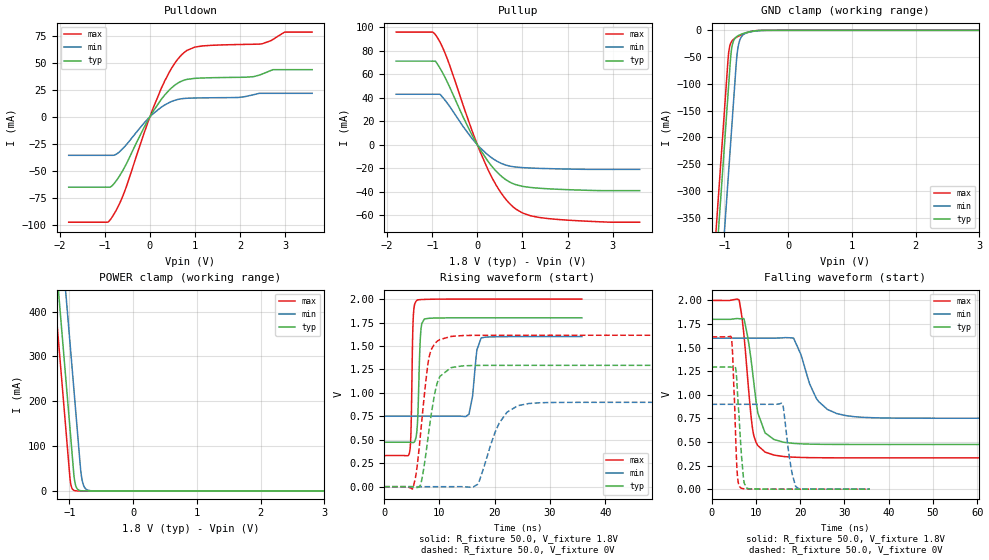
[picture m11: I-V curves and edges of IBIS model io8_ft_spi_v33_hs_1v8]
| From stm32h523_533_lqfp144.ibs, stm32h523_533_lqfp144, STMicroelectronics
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[Model]   io8_ft_spi_v33_hs_1v8
Model_type I/O
Polarity   Non-Inverting
Enable   Active-Low
| CAP_THRESHOLD on pad IOFT is "UDTCAPC" :
| Rising=20.0% of vddiom   Falling=80.0% of vddiom
| C_comp min and max val. don't necessarily correlate with the min and max pvt
| but are the smallest and greatest pad capacitance found.
| var   typ   min   max
C_comp   3.69208pF  3.66960pF  3.86716pF
|C_comp_pullup   2.28930pF  2.21680pF  2.21510pF
|C_comp_pulldown   1.40278pF  1.45280pF  1.65206pF
Vinl = 480.0mV
Vinh = 1.4V
Vmeas = 900.0mV   | Reference voltage for timing measurements
Cref  = 50.0pF   | Timing specification test load capacitance value
Rref  = 100.0MOhm   | Timing specification test load resistance value
Vref  = 900.0mV   | Timing specification test load voltage
[Model Spec]
| TIME_THRESHOLD on pin ZIV33M is "CMOS" :
| Rising=40.0% of vddiom   Falling=60.0% of vddiom
Vinl 693.80000mV 621.80000mV 774.80000mV
Vinh 1.05820V 933.20000mV 1.16320V
| variable   typ   min   max
[Temperature Range] 25.0 125.0 -40.0
| variable   typ   min   max
[Voltage Range] 1.8V 1.6V 2.0V
| variable   typ   min   max
[POWER Clamp Reference] 1.8V 1.6V 2.0V
| variable   typ   min   max
[GND Clamp Reference] 0V 0V 0V
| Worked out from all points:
|   slope of the pulldown table from 0 to 0.27 V, typ, clamps not added: 15.8 ohm
|   slope of the pullup table from 0 to 0.27 V, typ, clamps not added: 17.1 ohm
|   GND clamp passes 1 mA (typ) near -0.52 V on its own axis
|   POWER clamp passes 1 mA (typ) near -0.84 V on its own axis
|   rising waveform, R_fixture 50.0, V_fixture 1.8V: 20-80 % time 426ps typ, 879ps min, 294ps max; typ from 0.474 V to 1.8 V
|   falling waveform, R_fixture 50.0, V_fixture 1.8V: 20-80 % time 2.56ns typ, 4.2ns min, 1.95ns max; typ from 1.8 V to 0.474 V
|   rising waveform, R_fixture 50.0, V_fixture 0V: 20-80 % time 1.97ns typ, 3.43ns min, 1.71ns max; typ from 0 V to 1.29 V
|   falling waveform, R_fixture 50.0, V_fixture 0V: 20-80 % time 1.1ns typ, 1.55ns min, 755ps max; typ from 1.29 V to 0 V
[POWER Clamp]
-1.8V     1.518A     1.709A     1.407A
-1.23V    548.8mA    740.2mA    437.5mA
-1.16V    429.8mA    621.2mA    318.5mA
-1.05V    242.8mA    434.2mA    131.5mA
-980mV    123.8mA    315.2mA    17.95mA
-930mV    38.81mA    230.2mA    1.49mA
-910mV    17.82mA    196.2mA    550.8uA
-890mV    8.18mA     162.2mA    203.5uA
-810mV    363.5uA    33.6mA     3.797uA
-770mV    76.62uA    10.47mA    518.8nA
-710mV    7.416uA    1.822mA    26.34nA
3.6V      0A         0A         0A
[GND Clamp]
-1.8V     -1.579A    -1.74A     -1.515A
-1.24V    -627.3mA   -788.3mA   -562.7mA
-1.05V    -304.3mA   -465.3mA   -239.7mA
-940mV    -117.3mA   -278.3mA   -52.69mA
-930mV    -100.3mA   -261.3mA   -40.52mA
-900mV    -50.11mA   -210.3mA   -24.23mA
-880mV    -30.95mA   -176.3mA   -20.02mA
-810mV    -12.18mA   -57.97mA   -13.23mA
-780mV    -9.807mA   -29.1mA    -11.19mA
-690mV    -5.41mA    -7.142mA   -6.184mA
-420mV    -170.4uA   -446.1uA   -81.94uA
3.6V      5.755nA    953.4nA    228.2pA
| variable   typ   min   max
[Pullup Reference] 1.8V 1.6V 2.0V
| variable   typ   min   max
[Pulldown Reference] 0V 0V 0V
[Pullup]
-1.8V     71.25mA    43.04mA    95.97mA
-990mV    71.25mA    43.04mA    95.97mA
-900mV    69.58mA    43.04mA    92.06mA
-830mV    65.3mA     43.04mA    87.53mA
-670mV    53.67mA    35.6mA     73.46mA
-120mV    8.372mA    5.391mA    12.2mA
220mV     -13.2mA    -8.17mA    -19.85mA
520mV     -26.34mA   -15.62mA   -40.64mA
820mV     -33.51mA   -18.79mA   -53.71mA
1.18V     -36.34mA   -19.79mA   -60.45mA
1.56V     -37.44mA   -20.28mA   -62.79mA
3.6V      -39.03mA   -20.93mA   -65.9mA
[Pulldown]
-1.8V     -65.02mA   -35.56mA   -97.42mA
-940mV    -65.02mA   -35.56mA   -97.42mA
-850mV    -64.17mA   -35.56mA   -93.49mA
-570mV    -47.32mA   -28.01mA   -70.04mA
-120mV    -9.088mA   -5.279mA   -14.07mA
250mV     16.04mA    8.832mA    26.05mA
520mV     28.19mA    14.82mA    47.53mA
780mV     34.17mA    17.07mA    60.14mA
1.18V     35.97mA    17.56mA    65.65mA
2.49V     39.57mA    21.77mA    67.55mA
2.99V     43.62mA    21.77mA    78.38mA
3.6V      43.62mA    21.77mA    78.38mA
[Ramp]
dV/dt_r 776.15655mV/1.97139ns 539.54478mV/3.32002ns 968.54221mV/1.70584ns
dV/dt_f 795.78722mV/2.30829ns 508.982mV/4.15348ns 1.00099V/1.94881ns
R_load = 50.0
| Removed startup time: 0s 0s 0s  .
| Removed end time: 35.75ns.
[Rising Waveform]
R_fixture   = 50.0
V_fixture   = 1.8V
V_fixture_min = 1.6V
V_fixture_max = 2.0V
0s        473.7mV    751.7mV    331.7mV
4.6ns     473.7mV    751.7mV    361.3mV
4.85ns    472.9mV    751.7mV    544.7mV
5.3ns     470.8mV    751.7mV    1.823V
5.95ns    602mV      751.7mV    1.986V
6.6ns     1.619V     751.7mV    1.994V
7.3ns     1.788V     751.7mV    1.996V
15.35ns   1.8V       771.8mV    2V
17.55ns   1.8V       1.586V     2V
35.75ns   1.8V       1.6V       2V
| Removed startup time: 0s 0s 0s  .
| Removed end time: 98.75ns.
[Falling Waveform]
R_fixture   = 50.0
V_fixture   = 1.8V
V_fixture_min = 1.6V
V_fixture_max = 2.0V
0s        1.8V       1.6V       2V
6.25ns    1.806V     1.6V       2.001V
7.4ns     1.791V     1.6V       1.595V
9.35ns    1.211V     1.6V       617mV
10.45ns   809.1mV    1.6V       462.4mV
12.1ns    596.1mV    1.6V       393.1mV
18.55ns   485.2mV    1.599V     339mV
23.65ns   476mV      964.2mV    333.4mV
30.25ns   474mV      780.1mV    332mV
98.75ns   473.7mV    751.7mV    331.7mV
| Removed startup time: 0s 0s 0s  .
| Removed end time: 98.6ns.
[Rising Waveform]
R_fixture   = 50.0
V_fixture   = 0V
V_fixture_min = 0V
V_fixture_max = 0V
0s        180.2nV    440.2nV    129.4nV
5.2ns     -1.058mV   447.5nV    -19.21mV
6.7ns     40.84mV    449.7nV    624.9mV
8.2ns     634mV      454.6nV    1.395V
9.8ns     1.137V     433.9nV    1.558V
12.1ns    1.269V     1.052uV    1.602V
16.9ns    1.292V     24.37mV    1.613V
20.8ns    1.293V     676mV      1.614V
26.2ns    1.294V     886.8mV    1.614V
98.6ns    1.294V     899.2mV    1.614V
| Removed startup time: 0s 0s 0s  .
| Removed end time: 35.75ns.
[Falling Waveform]
R_fixture   = 50.0
V_fixture   = 0V
V_fixture_min = 0V
V_fixture_max = 0V
0s        1.294V     899.3mV    1.614V
4.45ns    1.293V     899.3mV    1.611V
5.8ns     1.078V     899.3mV    175.5mV
6.6ns     470.8mV    899.3mV    13.92mV
7.3ns     88.68mV    899.3mV    4.365mV
8.05ns    7.755mV    899.3mV    2.245mV
16.05ns   213.3uV    899mV      156.1uV
18.25ns   107.5uV    155.8mV    84.52uV
19.75ns   68.1uV     5.173mV    55.32uV
35.75ns   527.1nV    97.63uV    581.2nV
